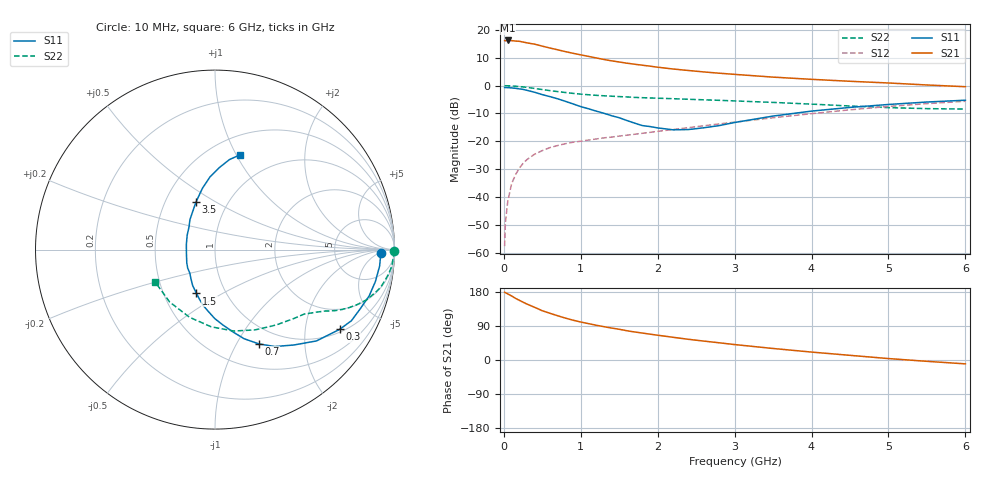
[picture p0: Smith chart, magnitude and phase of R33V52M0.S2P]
! SIEMENS Small Signal Semiconductors
! BFR181
! Si NPN RF Bipolar Junction Transistor in SOT23
! VCE = 3.5 V  IC = 2 mA
! Common Emitter S-Parameters:  May  1996
# GHz  S  MA  R  50
!  f  S11  S21  S12  S22
! GHz  MAG  ANG  MAG  ANG  MAG  ANG  MAG  ANG
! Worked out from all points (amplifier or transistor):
!   36 points, 10 MHz to 6 GHz, reference 50 ohm
!   highest |S21| = 16.3 dB at 50 MHz (marker M1)
!   |S21| within 3 dB of that: start of sweep to 643.3 MHz
!   unconditionally stable (mu >= 1): 1.606 GHz to 3.367 GHz
!   at 250 MHz: K = 0.23, MSG = 21.8 dB, |S12| = -28.0 dB
!   at 1.4 GHz: K = 0.94, MSG = 13.7 dB, |S12| = -18.5 dB
!   at 6 GHz: K = 0.86, MSG = 2.6 dB, |S12| = -5.6 dB
!   lowest NFmin = 1.35 dB at 450 MHz
!   S11 on the Smith chart (normalised r, x): 10 MHz: 24, -6; 300 MHz: 1.10, -3.07; 700 MHz: 0.78, -1.24; 1.5 GHz: 0.73, -0.38; 3.5 GHz: 0.71, +0.41; 6 GHz: 0.69, +1.04
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0.01  0.9249 -1.2  6.463 179.0  0.0013 90.7  0.997 -0.5
0.02  0.9234 -2.1  6.386 177.6  0.0034 80.9  0.9964 -1.1
0.05  0.9218 -5.7  6.494 174.5  0.0081 86.0  0.9946 -2.6
0.1  0.9111 -11.3  6.449 169.2  0.0171 83.2  0.9893 -5.3
0.15  0.8969 -16.7  6.334 162.9  0.0248 79.2  0.9775 -7.9
0.2  0.8741 -22.1  6.275 157.7  0.0327 76.6  0.963 -10.2
0.3  0.8254 -32.5  5.878 147.6  0.0468 71.3  0.93 -14.5
0.4  0.7605 -42.0  5.572 139.0  0.0586 66.5  0.8914 -18.2
0.5  0.6897 -50.4  5.133 130.0  0.068 62.9  0.85 -21.1
0.7  0.5799 -65.0  4.411 116.7  0.0839 57.6  0.7817 -25.3
0.8  0.5225 -71.9  4.09 110.6  0.0904 55.7  0.7532 -26.8
0.9  0.4695 -77.7  3.818 105.0  0.0961 54.5  0.726 -28.1
1.1  0.3843 -90.2  3.359 96.0  0.1051 53.5  0.686 -30.2
1.3  0.3191 -101.7  2.959 88.0  0.115 53.2  0.6571 -32.1
1.5  0.2649 -112.9  2.665 81.1  0.1239 53.5  0.6353 -33.9
1.8  0.1915 -137.3  2.33 71.1  0.1391 54.6  0.6076 -36.7
2.2  0.1607 -172.4  1.993 59.9  0.1626 55.6  0.5823 -41.4
2.8  0.1915 139.2  1.674 45.4  0.2051 55.8  0.5448 -49.8
3.5  0.2839 112.1  1.423 30.4  0.2649 53.3  0.4996 -63.6
4.5  0.4061 93.9  1.198 12.3  0.3679 45.3  0.4306 -92.9
5.5  0.5077 80.9  1.028 -3.5  0.4751 32.8  0.3861 -131.0
6  0.5473 75.1  0.957 -10.2  0.5238 25.4  0.3791 -151.6
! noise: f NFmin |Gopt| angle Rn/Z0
0.45  1.35  0.6  17  0.4
0.9  1.45  0.5  36  0.4
1.8  1.8  0.31  80  0.37
